(* Logix 5000 AddOnInstructionDefinition export B256_StoC; software revision 30.00 *)

ADD_ON_INSTRUCTION D_SHL   (* revision 1.0, vendor Ken Fischer, NSWCPD, C512 *)
// DINT bit shift left of the 32-bit argument Inp_A by Inp_B bits with paddding by zeros on the right
// Revision note:
// Rev1.0: TBD - Initial Release
VAR_IN_OUT
   Inp_A : DINT; {required}   // 64-bit Integer to be right circular rotated
END_VAR
VAR_INPUT
   Inp_B : INT; {required}   // Number of bits to shift
END_VAR
VAR_IN_OUT
   Out : DINT; {required}   // Result
END_VAR
VAR
   Wrk_InpA : DINT[2];
   Source_Bit : BOOL;
   ONS : BOOL;
   BSL_Cntrl : CONTROL := (LEN := 32);
END_VAR

ROUTINE Logic   (* ladder *)
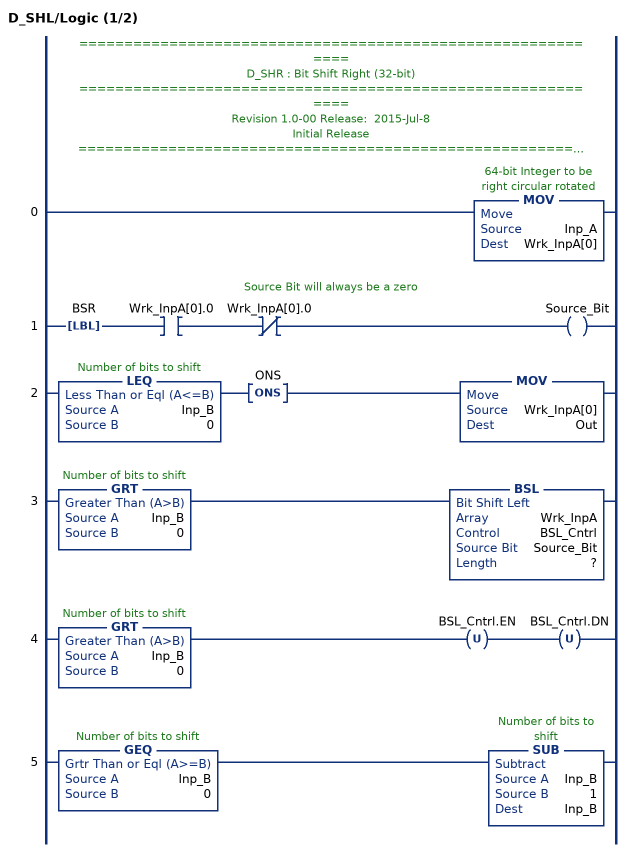
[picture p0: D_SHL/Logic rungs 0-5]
   // ============================================================
   // D_SHR : Bit Shift Right (32-bit)
   // ============================================================
   // Revision 1.0-00 Release:  2015-Jul-8
   // Initial Release
   // ============================================================
   // Performs a left bit shift of the 32-bit argument Inp_A by the
   // number of bits defined in the 16-bit argument Inp_B, with padding by zeros.
   0: MOV(Inp_A,Wrk_InpA[0]);
   // Source Bit will always be a zero
   1: LBL(BSR)XIC(Wrk_InpA[0].0)XIO(Wrk_InpA[0].0)OTE(Source_Bit);
   2: LEQ(Inp_B,0)ONS(ONS)MOV(Wrk_InpA[0],Out);
   3: GRT(Inp_B,0)BSL(Wrk_InpA,BSL_Cntrl,Source_Bit,?);
   4: GRT(Inp_B,0)OTU(BSL_Cntrl.EN)OTU(BSL_Cntrl.DN);
   5: GEQ(Inp_B,0)SUB(Inp_B,1,Inp_B);
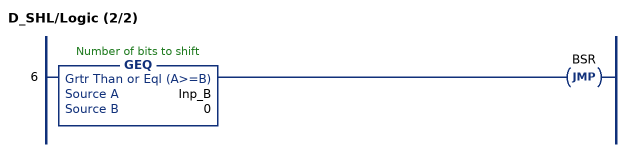
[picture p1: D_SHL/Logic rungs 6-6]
   6: GEQ(Inp_B,0)JMP(BSR);
END_ROUTINE
END_ADD_ON_INSTRUCTION

ADD_ON_INSTRUCTION B256_StoC   (* revision 1.0 20170916, vendor Kenneth A. Fischer *)
// Convert 256-bit value using 64 hex string characters into 256-bit value using 22 12-bit pieces
// Revision note:
// Rev1.0: 20170916 - Initial Release
VAR_IN_OUT
   Inp_S : STRING; {required}
   Out_C : DINT[22]; {required}
END_VAR
VAR
   byte : DINT[3];
   D_SHL : D_SHL;
   i : INT;
   j : INT;
   k : DINT;
   temp : DINT;
END_VAR

ROUTINE Logic   (* ladder *)
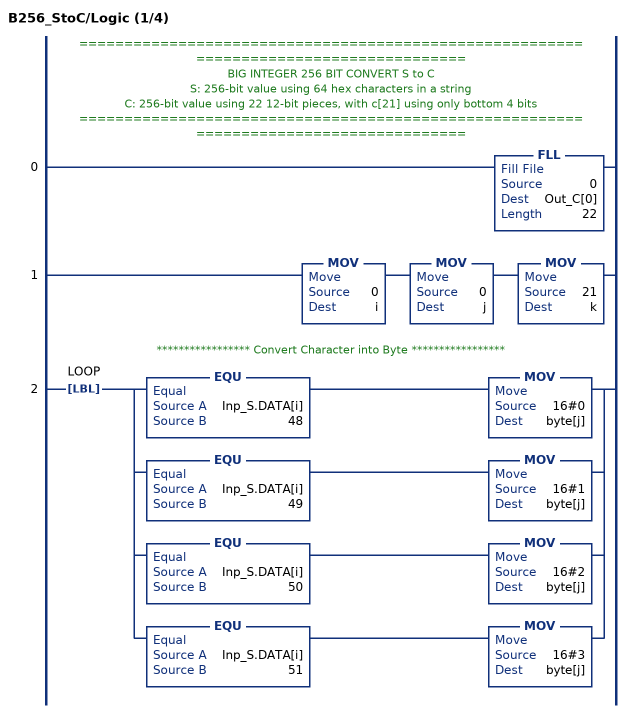
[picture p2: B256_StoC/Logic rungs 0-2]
   // ======================================================================================
   // BIG INTEGER 256 BIT CONVERT S to C
   // S: 256-bit value using 64 hex characters in a string
   // C: 256-bit value using 22 12-bit pieces, with c[21] using only bottom 4 bits
   // ======================================================================================
   0: FLL(0,Out_C[0],22);
   1: MOV(0,i)MOV(0,j)MOV(21,k);
   // ***************** Convert Character into Byte *****************
   2: LBL(LOOP)[EQU(Inp_S.DATA[i],48) MOV(16#0,byte[j]) ,EQU(Inp_S.DATA[i],49) MOV(16#1,byte[j]) ,EQU(Inp_S.DATA[i],50) MOV(16#2,byte[j]) ,EQU(Inp_S.DATA[i],51) MOV(16#3,byte[j]) ];
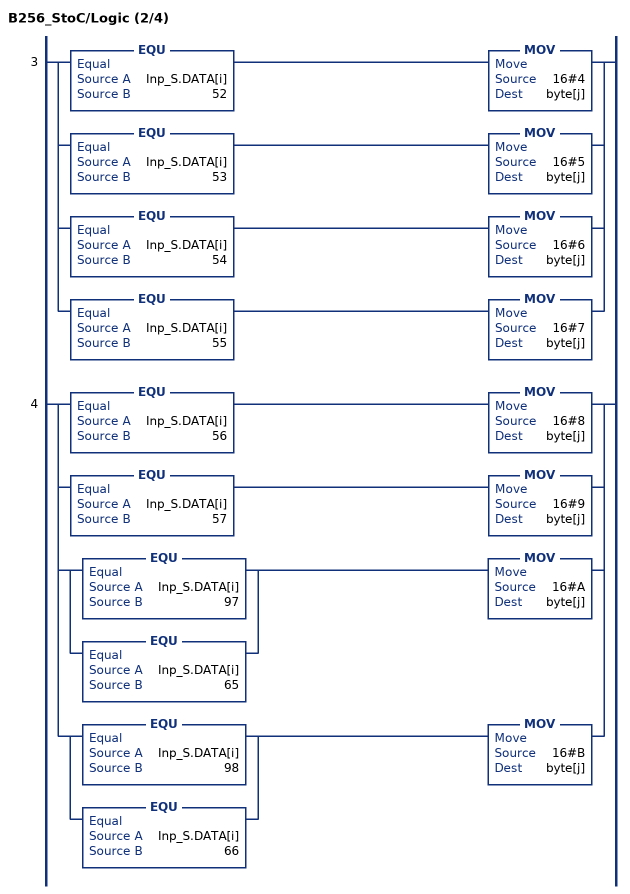
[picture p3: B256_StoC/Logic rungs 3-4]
   3: [EQU(Inp_S.DATA[i],52) MOV(16#4,byte[j]) ,EQU(Inp_S.DATA[i],53) MOV(16#5,byte[j]) ,EQU(Inp_S.DATA[i],54) MOV(16#6,byte[j]) ,EQU(Inp_S.DATA[i],55) MOV(16#7,byte[j]) ];
   4: [EQU(Inp_S.DATA[i],56) MOV(16#8,byte[j]) ,EQU(Inp_S.DATA[i],57) MOV(16#9,byte[j]) ,[EQU(Inp_S.DATA[i],97) ,EQU(Inp_S.DATA[i],65) ] MOV(16#A,byte[j]) ,[EQU(Inp_S.DATA[i],98) ,EQU(Inp_S.DATA[i],66) ] MOV(16#B,byte[j]) ];
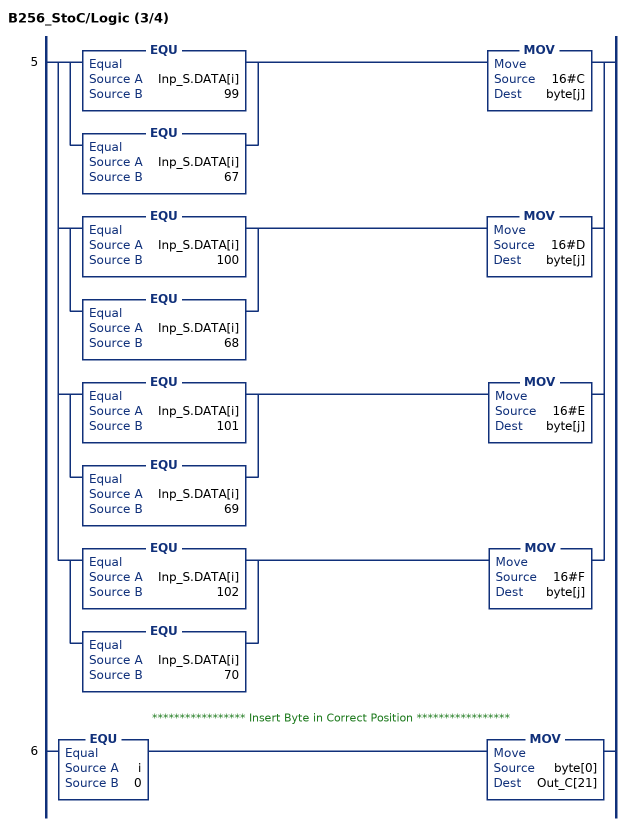
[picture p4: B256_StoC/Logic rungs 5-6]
   5: [[EQU(Inp_S.DATA[i],99) ,EQU(Inp_S.DATA[i],67) ] MOV(16#C,byte[j]) ,[EQU(Inp_S.DATA[i],100) ,EQU(Inp_S.DATA[i],68) ] MOV(16#D,byte[j]) ,[EQU(Inp_S.DATA[i],101) ,EQU(Inp_S.DATA[i],69) ] MOV(16#E,byte[j]) ,[EQU(Inp_S.DATA[i],102) ,EQU(Inp_S.DATA[i],70) ] MOV(16#F,byte[j]) ];
   // ***************** Insert Byte in Correct Position *****************
   6: EQU(i,0)MOV(byte[0],Out_C[21]);
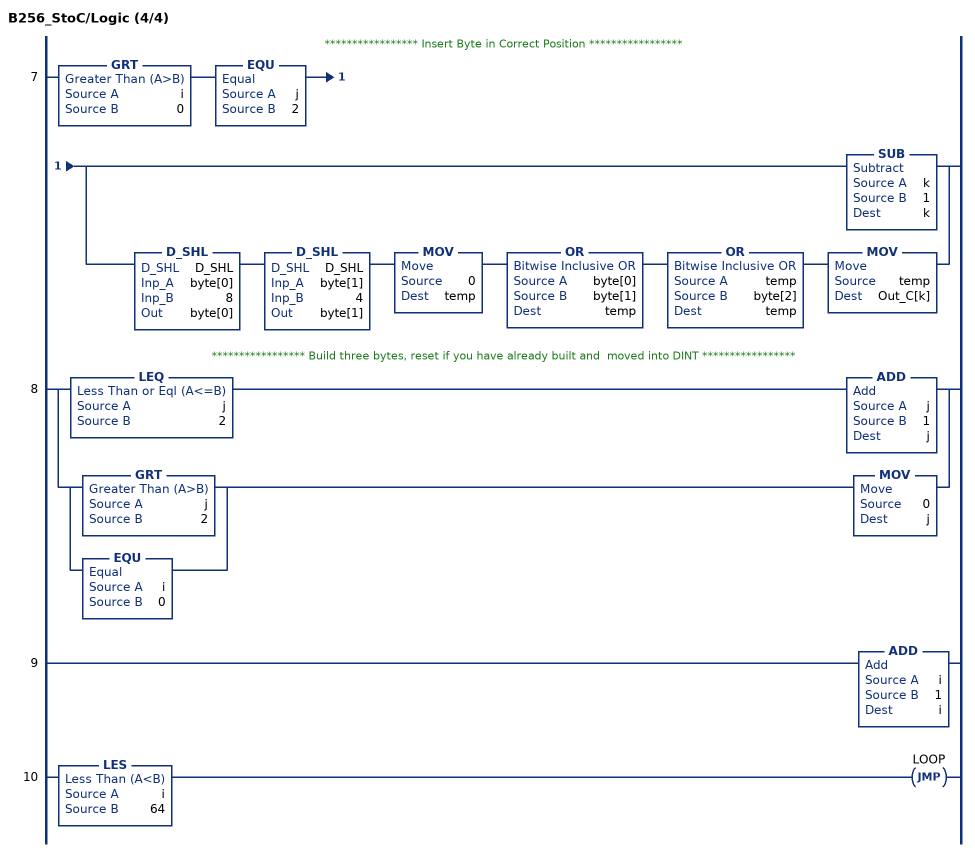
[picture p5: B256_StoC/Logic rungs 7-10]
   // ***************** Insert Byte in Correct Position *****************
   7: GRT(i,0)EQU(j,2)[SUB(k,1,k) ,D_SHL(D_SHL,byte[0],8,byte[0]) D_SHL(D_SHL,byte[1],4,byte[1]) MOV(0,temp) OR(byte[0],byte[1],temp) OR(temp,byte[2],temp) MOV(temp,Out_C[k]) ];
   // ***************** Build three bytes, reset if you have already built and  moved into DINT *****************
   8: [LEQ(j,2) ADD(j,1,j) ,[GRT(j,2) ,EQU(i,0) ] MOV(0,j) ];
   9: ADD(i,1,i);
   10: LES(i,64)JMP(LOOP);
END_ROUTINE
END_ADD_ON_INSTRUCTION
